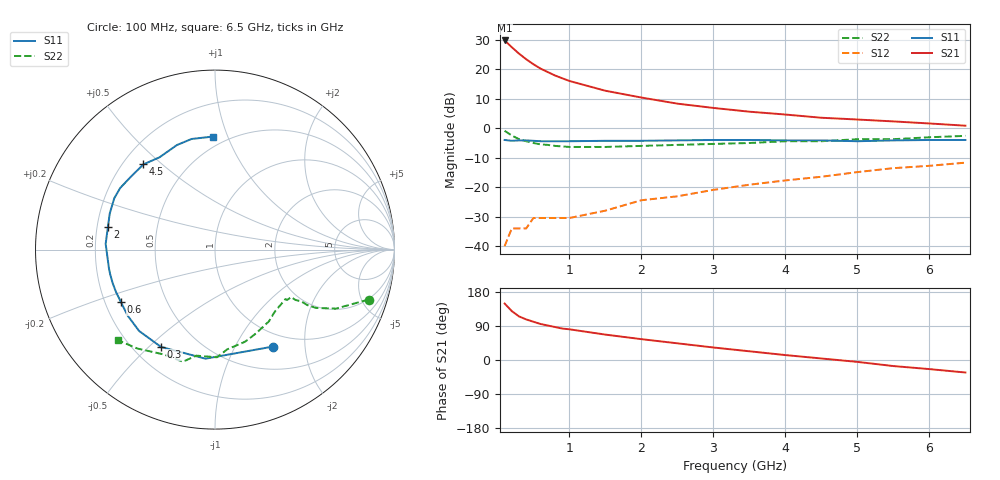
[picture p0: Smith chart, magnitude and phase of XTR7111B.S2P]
! HXTR-7111 Common Emitter
! Vce=15V  Ic=18mA
# ghz s ma r 50
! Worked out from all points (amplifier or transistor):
!   21 points, 100 MHz to 6.5 GHz, reference 50 ohm
!   highest |S21| = 29.7 dB at 100 MHz (marker M1)
!   |S21| within 3 dB of that: start of sweep to 232.5 MHz
!   unconditionally stable (mu >= 1): 904.3 MHz to 1.962 GHz; 2.291 GHz to 2.538 GHz
!   at 400 MHz: K = 0.56, MSG = 28.7 dB, |S12| = -34.0 dB
!   at 1.5 GHz: K = 1.20, MAG = 17.6 dB, |S12| = -28.0 dB
!   at 6.5 GHz: K = 0.34, MSG = 6.3 dB, |S12| = -11.7 dB
!   S11 on the Smith chart (normalised r, x): 100 MHz: 0.81, -1.44; 300 MHz: 0.31, -0.55; 600 MHz: 0.27, -0.24; 2 GHz: 0.24, +0.10; 4.5 GHz: 0.28, +0.44; 6.5 GHz: 0.43, +0.89
0.1  0.63 -59.0  30.6 149.0  0.01 64.0  0.9 -18.0
0.2  0.61 -95.0  23.5 129.0  0.02 46.0  0.75 -26.0
0.3  0.62 -119.0  18.3 115.0  0.02 48.0  0.65 -30.0
0.4  0.62 -133.0  14.7 107.0  0.02 43.0  0.6 -31.0
0.5  0.61 -143.0  12.1 101.0  0.03 48.0  0.56 -31.0
0.6  0.6 -151.0  10.2 95.0  0.03 44.0  0.53 -32.0
0.7  0.6 -157.0  8.9 91.0  0.03 49.0  0.52 -32.0
0.8  0.6 -162.0  7.8 87.0  0.03 49.0  0.5 -32.0
0.9  0.6 -167.0  7 83.0  0.03 51.0  0.49 -35.0
1  0.6 -170.0  6.3 81.0  0.03 51.0  0.48 -35.0
1.5  0.61 177.0  4.3 67.0  0.04 60.0  0.48 -46.0
2  0.61 168.0  3.3 55.0  0.06 65.0  0.5 -53.0
2.5  0.62 161.0  2.6 44.0  0.07 67.0  0.52 -64.0
3  0.63 153.0  2.2 33.0  0.09 68.0  0.54 -72.0
3.5  0.63 147.0  1.9 23.0  0.11 66.0  0.56 -83.0
4  0.62 139.0  1.7 13.0  0.13 64.0  0.6 -89.0
4.5  0.62 130.0  1.5 4.0  0.15 60.0  0.6 -100.0
5  0.6 121.0  1.4 -5.0  0.18 56.0  0.65 -106.0
5.5  0.62 110.0  1.3 -16.0  0.21 52.0  0.65 -116.0
6  0.63 102.0  1.2 -24.0  0.23 46.0  0.7 -128.0
6.5  0.63 91.0  1.1 -33.0  0.26 40.0  0.74 -137.0
